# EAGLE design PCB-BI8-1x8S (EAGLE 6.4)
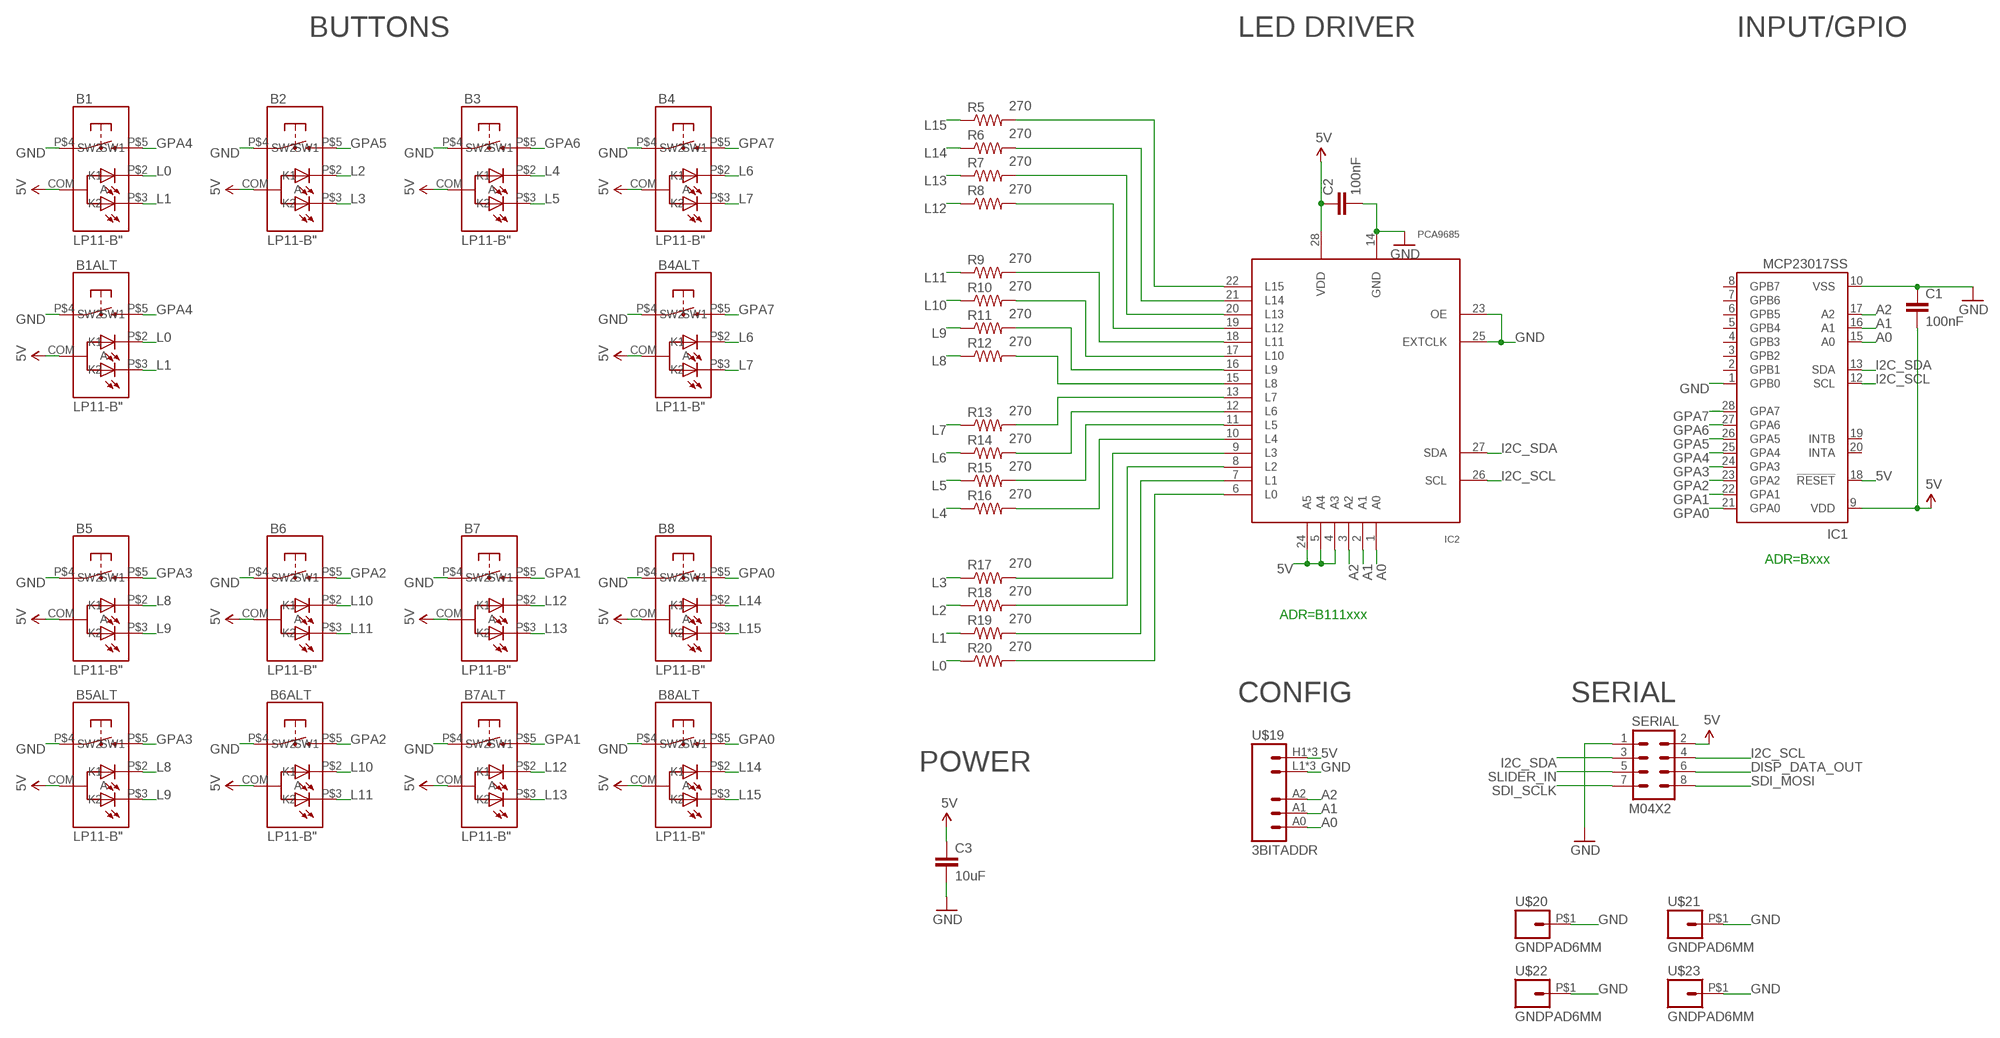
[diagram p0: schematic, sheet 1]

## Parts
B1  LP11-B"  [LP11]
B1ALT  LP11-B"  [LP11]
B2  LP11-B"  [LP11]
B3  LP11-B"  [LP11]
B4  LP11-B"  [LP11]
B4ALT  LP11-B"  [LP11]
B5  LP11-B"  [LP11]
B5ALT  LP11-B"  [LP11]
B6  LP11-B"  [LP11]
B6ALT  LP11-B"  [LP11]
B7  LP11-B"  [LP11]
B7ALT  LP11-B"  [LP11]
B8  LP11-B"  [LP11]
B8ALT  LP11-B"  [LP11]
C1  100nF  CAP0603-CAP  [0603-CAP]
C2  100nF  CAP0603-CAP  [0603-CAP]
C3  10uF  CAP0805  [0805]
IC1  MCP23017SS  [SSOP28]
IC2  PCA9685  [TSSOP28]
R5  270  RESISTOR0603-RES  [0603-RES]
R6  270  RESISTOR0603-RES  [0603-RES]
R7  270  RESISTOR0603-RES  [0603-RES]
R8  270  RESISTOR0603-RES  [0603-RES]
R9  270  RESISTOR0603-RES  [0603-RES]
R10  270  RESISTOR0603-RES  [0603-RES]
R11  270  RESISTOR0603-RES  [0603-RES]
R12  270  RESISTOR0603-RES  [0603-RES]
R13  270  RESISTOR0603-RES  [0603-RES]
R14  270  RESISTOR0603-RES  [0603-RES]
R15  270  RESISTOR0603-RES  [0603-RES]
R16  270  RESISTOR0603-RES  [0603-RES]
R17  270  RESISTOR0603-RES  [0603-RES]
R18  270  RESISTOR0603-RES  [0603-RES]
R19  270  RESISTOR0603-RES  [0603-RES]
R20  270  RESISTOR0603-RES  [0603-RES]
SERIAL  M04X2  [2X4]
U$19  3BITADDR  [3BITADDR]
U$20  GNDPAD6MM  [3.2MMPAD6MM]
U$21  GNDPAD6MM  [3.2MMPAD6MM]
U$22  GNDPAD6MM  [3.2MMPAD6MM]
U$23  GNDPAD6MM  [3.2MMPAD6MM]

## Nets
5V [Power]: B1.COM(A) B1ALT.COM(A) B2.COM(A) B3.COM(A) B4.COM(A) B4ALT.COM(A) B5.COM(A) B5ALT.COM(A) B6.COM(A) B6ALT.COM(A) B7.COM(A) B7ALT.COM(A) B8.COM(A) B8ALT.COM(A) C1.2 C2.1 C3.1 IC1.9(VDD) IC1.18(!RESET) IC2.4(A3) IC2.5(A4) IC2.24(A5) IC2.28(VDD) SERIAL.2 U$19.H1(VCC) U$19.H2(VCC) U$19.H3(VCC)
A0: IC1.15(A0) IC2.1(A0) U$19.A0
A1: IC1.16(A1) IC2.2(A1) U$19.A1
A2: IC1.17(A2) IC2.3(A2) U$19.A2
DISP_DATA_OUT: SERIAL.6
GND [Power]: B1.P$4(SW1) B1ALT.P$4(SW1) B2.P$4(SW1) B3.P$4(SW1) B4.P$4(SW1) B4ALT.P$4(SW1) B5.P$4(SW1) B5ALT.P$4(SW1) B6.P$4(SW1) B6ALT.P$4(SW1) B7.P$4(SW1) B7ALT.P$4(SW1) B8.P$4(SW1) B8ALT.P$4(SW1) C1.1 C2.2 C3.2 IC1.1(GPB0) IC1.10(VSS) IC2.14(GND) IC2.23(OE) IC2.25(EXTCLK) SERIAL.1 U$19.L1(GND) U$19.L2(GND) U$19.L3(GND) U$20.P$1 U$21.P$1 U$22.P$1 U$23.P$1
GPA0: B8.P$5(SW2) B8ALT.P$5(SW2) IC1.21(GPA0)
GPA1: B7.P$5(SW2) B7ALT.P$5(SW2) IC1.22(GPA1)
GPA2: B6.P$5(SW2) B6ALT.P$5(SW2) IC1.23(GPA2)
GPA3: B5.P$5(SW2) B5ALT.P$5(SW2) IC1.24(GPA3)
GPA4: B1.P$5(SW2) B1ALT.P$5(SW2) IC1.25(GPA4)
GPA5: B2.P$5(SW2) IC1.26(GPA5)
GPA6: B3.P$5(SW2) IC1.27(GPA6)
GPA7: B4.P$5(SW2) B4ALT.P$5(SW2) IC1.28(GPA7)
I2C_SCL: IC1.12(SCL) IC2.26(SCL) SERIAL.4
I2C_SDA: IC1.13(SDA) IC2.27(SDA) SERIAL.3
L0: B1.P$2(K1) B1ALT.P$2(K1) R20.1
L1: B1.P$3(K2) B1ALT.P$3(K2) R19.1
L2: B2.P$2(K1) R18.1
L3: B2.P$3(K2) R17.1
L4: B3.P$2(K1) R16.1
L5: B3.P$3(K2) R15.1
L6: B4.P$2(K1) B4ALT.P$2(K1) R14.1
L7: B4.P$3(K2) B4ALT.P$3(K2) R13.1
L8: B5.P$2(K1) B5ALT.P$2(K1) R12.1
L9: B5.P$3(K2) B5ALT.P$3(K2) R11.1
L10: B6.P$2(K1) B6ALT.P$2(K1) R10.1
L11: B6.P$3(K2) B6ALT.P$3(K2) R9.1
L12: B7.P$2(K1) B7ALT.P$2(K1) R8.1
L13: B7.P$3(K2) B7ALT.P$3(K2) R7.1
L14: B8.P$2(K1) B8ALT.P$2(K1) R6.1
L15: B8.P$3(K2) B8ALT.P$3(K2) R5.1
N$4: IC2.13(L7) R13.2
N$5: IC2.12(L6) R14.2
N$7: IC2.11(L5) R15.2
N$9: IC2.10(L4) R16.2
N$10: IC2.9(L3) R17.2
N$11: IC2.8(L2) R18.2
N$12: IC2.7(L1) R19.2
N$19: IC2.6(L0) R20.2
N$20: IC2.15(L8) R12.2
N$21: IC2.16(L9) R11.2
N$22: IC2.17(L10) R10.2
N$23: IC2.18(L11) R9.2
N$24: IC2.19(L12) R8.2
N$25: IC2.20(L13) R7.2
N$26: IC2.21(L14) R6.2
N$27: IC2.22(L15) R5.2
SDI_MOSI: SERIAL.8
SDI_SCLK: SERIAL.7
SLIDER_IN: SERIAL.5
Unconnected: IC1.2(GPB1) IC1.3(GPB2) IC1.4(GPB3) IC1.5(GPB4) IC1.6(GPB5) IC1.7(GPB6) IC1.8(GPB7) IC1.19(INTB) IC1.20(INTA)

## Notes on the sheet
- BUTTONS | LED DRIVER | INPUT/GPIO
- ADR=Bxxx
- ADR=B111xxx
- CONFIG | SERIAL
- POWER

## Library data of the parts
B1 B1ALT B2-B4 B4ALT B5 B5ALT B6 B6ALT B7 B7ALT B8 B8ALT = SKAARHOJ:LP11-B
C1-C3 = SparkFun:CAP: Capacitor
IC1 = microchip:MCP23017: http://ww1.microchip.com/downloads/en/DeviceDoc/21952a.pdf Source: http://ww1.microchip.com/downloads/en/DeviceDoc/21952a.pdf; MF: MICROCHIP; MPN: MCP23017-E/SS; OC_FARNELL: 1467674; OC_NEWARK: 31K2960
IC2 = wsmith:PCA9685
R5-R20 = SparkFun:RESISTOR: Resistor
SERIAL = SparkFun:M04X2
U$19 = SKAARHOJ:3BITADDR
U$20-U$23 = SKAARHOJ:GNDPAD

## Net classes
0 default: width 0.203 mm, drill 0.305 mm, clearance 0.203 mm
1 Power: width 0.305 mm, drill 0.61 mm, clearance 0.203 mm

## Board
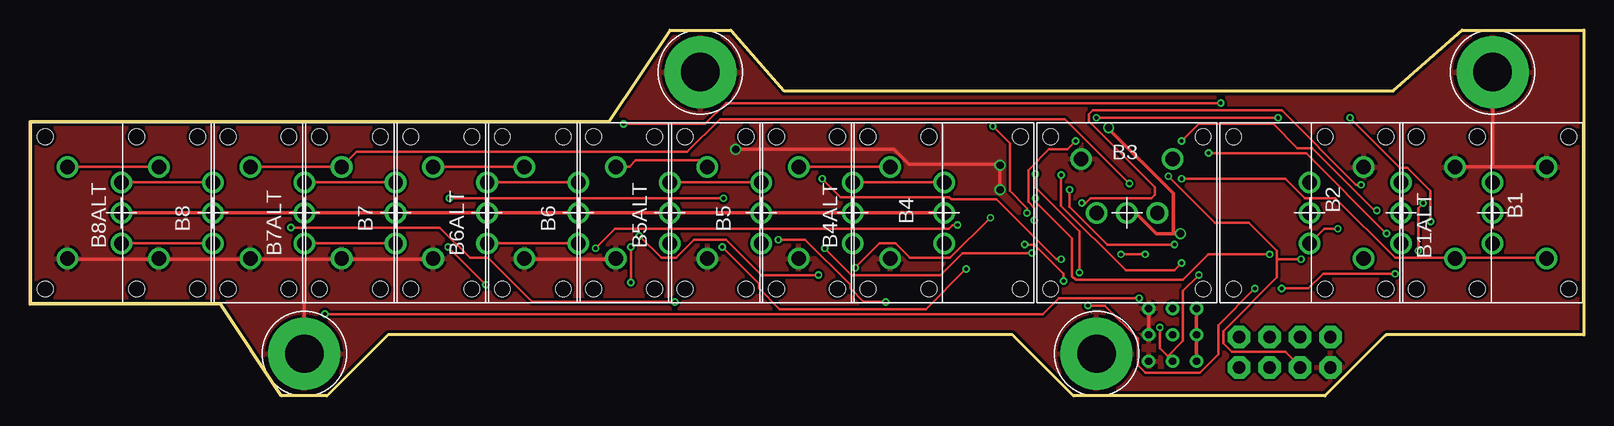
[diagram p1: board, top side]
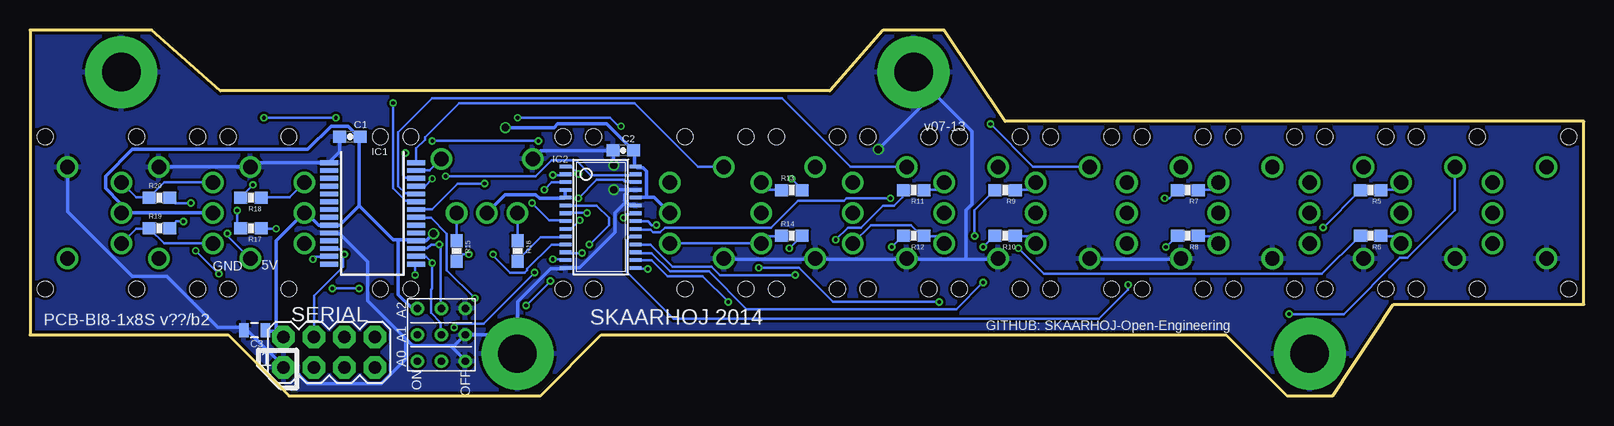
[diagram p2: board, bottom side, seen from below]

Size 129.54 x 30.48 mm. Coordinates in mm from the lower left corner, seen from the top.
Outline: 0,22.86 48.26,22.86 53.34,30.48 58.42,30.48 62.87,25.4 113.67,25.4 119.38,30.48 129.54,30.48 129.54,5.08 113.03,5.08 107.95,0 87,0 81.92,5.08 29.84,5.08 24.77,0 20.95,0 15.88,7.62 0,7.62 0,22.86
Copper layers (1*16): Top 0.035mm / dielectric 1.5mm / Bottom 0.035mm
Design rules "Fusion_eagle_rule_v1.1": minimum track width 6mil, minimum drill 12mil, track to track 6mil, track to pad 6mil, pad to pad 6mil, via to via 6mil, smd to smd 0mil, copper to edge 10mil, drill to drill 10mil, minimum pad ring 10mil, minimum via ring 6mil, stop-mask expansion 2mil, vias tented up to drill 100mil, thermal gap 10mil

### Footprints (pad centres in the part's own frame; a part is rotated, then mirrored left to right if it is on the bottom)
LP11 = drill 1.2: COM 0,0; P$2 0,2.54; P$3 0,-2.54; P$4 4.5,3.81; P$5 4.5,-3.81 | hole 1.3: -6.35,6.35; 6.35,6.35; 6.35,-6.35; -6.35,-6.35
0603-CAP = smd 1.1 x 1: 1 -0.85,0; 2 0.85,0
0805 = smd 0.8 x 1.2: 1 -0.9,0; 2 0.9,0
SSOP28 = smd 0.4 x 1.5: 1 -4.225,-3.625; 2 -3.575,-3.625; 3 -2.925,-3.625; 4 -2.275,-3.625; 5 -1.625,-3.625; 6 -0.975,-3.625; 7 -0.325,-3.625; 8 0.325,-3.625; 9 0.975,-3.625; 10 1.625,-3.625; 11 2.275,-3.625; 12 2.925,-3.625; 13 3.575,-3.625; 14 4.225,-3.625; 15 4.225,3.625; 16 3.575,3.625; 17 2.925,3.625; 18 2.275,3.625; 19 1.625,3.625; 20 0.975,3.625; 21 0.325,3.625; 22 -0.325,3.625; 23 -0.975,3.625; 24 -1.625,3.625; 25 -2.275,3.625; 26 -2.925,3.625; 27 -3.575,3.625; 28 -4.225,3.625
TSSOP28 = smd 0.305 x 0.991: 1 -4.225,-2.918; 2 -3.575,-2.918; 3 -2.925,-2.918; 4 -2.275,-2.918; 5 -1.625,-2.918; 6 -0.975,-2.918; 7 -0.325,-2.918; 8 0.325,-2.918; 9 0.975,-2.918; 10 1.625,-2.918; 11 2.275,-2.918; 12 2.925,-2.918; 13 3.575,-2.918; 14 4.225,-2.918; 15 4.225,2.918; 16 3.575,2.918; 17 2.925,2.918; 18 2.275,2.918; 19 1.625,2.918; 20 0.975,2.918; 21 0.325,2.918; 22 -0.325,2.918; 23 -0.975,2.918; 24 -1.625,2.918; 25 -2.275,2.918; 26 -2.925,2.918; 27 -3.575,2.918; 28 -4.225,2.918
0603-RES = smd 1.1 x 1: 1 -0.85,0; 2 0.85,0
2X4 = drill 1.016 pad 1.88 octagon: 1 -3.81,-1.27; 2 -3.81,1.27; 3 -1.27,-1.27; 4 -1.27,1.27; 5 1.27,-1.27; 6 1.27,1.27; 7 3.81,-1.27; 8 3.81,1.27
3BITADDR = drill 0.6: A0 -2.2,0; A1 0,0; A2 2.2,0; H1 -2.2,2; H2 0,2; H3 2.2,2; L1 -2.2,-2; L2 0,-2; L3 2.2,-2
3.2MMPAD6MM = drill 3.2 pad 6: P$1 0,0

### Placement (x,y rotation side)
B1  121.92,15.24 0 top
B1ALT  114.3,15.24 0 top
B2  106.68,15.24 0 top
B3  91.44,15.24 90 top
B4  76.2,15.24 180 top
B4ALT  68.58,15.24 180 top
B5  60.96,15.24 180 top
B5ALT  53.34,15.24 180 top
B6  45.72,15.24 180 top
B6ALT  38.1,15.24 180 top
B7  30.48,15.24 180 top
B7ALT  22.86,15.24 180 top
B8  15.24,15.24 180 top
B8ALT  7.62,15.24 180 top
C1  102.87,21.59 0 bottom
C2  80.09,20.45 180 bottom
C3  110.82,5.46 180 bottom
IC1  100.99,15.19 270 bottom
IC2  81.97,14.88 270 bottom
R5  17.78,17.14 180 bottom
R6  17.78,13.34 180 bottom
R7  33.02,17.14 180 bottom
R8  33.02,13.34 180 bottom
R9  48.26,17.14 180 bottom
R10  48.26,13.34 180 bottom
R11  55.88,17.14 180 bottom
R12  55.88,13.34 180 bottom
R13  66.04,17.14 0 bottom
R14  66.04,13.34 0 bottom
R15  93.98,12.06 270 bottom
R16  88.9,12.06 270 bottom
R17  111.12,13.97 180 bottom
R18  111.12,16.51 180 bottom
R19  118.75,13.97 0 bottom
R20  118.75,16.51 0 bottom
SERIAL  104.6,3.63 0 bottom
U$19  95.25,5.08 90 bottom
U$20  22.86,3.5 0 top
U$21  55.88,26.98 0 top
U$22  121.92,26.98 0 top
U$23  88.9,3.5 0 top

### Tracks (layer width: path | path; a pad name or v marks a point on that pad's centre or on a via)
5V  (via drill 0.61)
  Top 0.305: U$19.H1 97.23,2.95 97.23,5.08 U$19.H2 97.23,5.18 97.23,7.21 U$19.H3 | B3.COM 92.15,15.24 93.88,13.51 95.3,13.51 | v95.91,13.51 95.3,13.51 | B8ALT.COM B8.COM B7ALT.COM B7.COM B6ALT.COM B6.COM B5ALT.COM B5.COM B4ALT.COM B4.COM | 95.3,13.51 95.3,16.87 89.92,22.25 v89.92,22.35
  Bottom 0.305: B1ALT.COM B1.COM 122.02,15.34 122.02,16.05 123.24,17.27 123.24,18.29 121.01,20.52 106.38,20.52 104.44,22.45 103.02,22.45 102.21,21.64 C1.2 102.11,21.54 102.11,15.85 | IC2.4 84.94,17.07 84.94,16.56 IC2.5 85.04,16.46 87.07,16.46 87.38,16.76 89.92,16.76 B3.COM | C3.1 109.83,5.38 108.81,5.38 108.41,4.98 SERIAL.2 109.02,5.49 109.02,12.9 B2.COM 106.48,15.24 105.46,14.22 104.75,14.22 IC1.9 104.55,14.22 103.73,14.22 102.11,15.85 | 98.86,13.01 99.26,13.01 102.11,15.85 | 98.86,13.01 97.43,13.01 IC1.18 97.23,12.9 96.52,12.9 v95.91,13.51 | 98.86,13.01 98.86,8.43 97.74,7.32 97.33,7.32 U$19.H3 | 78.13,16.56 77.52,16.56 B4.COM | 78.13,16.56 79.05,16.56 IC2.24 | 78.13,16.56 78.13,18.69 78.44,19 78.94,19 IC2.28 79.15,19.2 79.15,20.42 C2.1 79.35,20.52 81.48,22.66 85.55,22.66 85.85,22.35 v89.92,22.35
A0  (via drill 0.3)
  Top 0.203: v83.82,18.49 83.82,17.37 87.48,13.72 v87.48,10.26 | v94.18,5.69 94.18,3.96 94.84,3.3 | 94.84,3.3 95.2,2.95 U$19.A0 | v97.43,10.06 96.11,8.74 96.11,4.57 94.84,3.3
  Bottom 0.203: v83.82,18.49 84.43,19.1 84.84,19.1 IC2.1 | v87.48,10.26 91.75,5.99 93.88,5.99 v94.18,5.69 | v97.43,10.06 97.43,10.87 IC1.15
A1  (via drill 0.3)
  Top 0.203: v85.95,18.39 85.95,15.85 91.34,10.46 95.4,10.46 v96.01,11.07
  Bottom 0.203: v85.95,18.39 84.94,18.39 IC2.2 | IC1.16 97.33,11.58 96.52,11.58 v96.01,11.07 96.01,8.94 96.11,8.84 96.11,6.91 95.3,6.1 95.3,5.08 U$19.A1
A2  (via drill 0.3)
  Top 0.203: v86.67,17.17 86.67,15.75 89.81,12.6 v95.4,12.6
  Bottom 0.203: v86.67,17.17 86.06,17.78 84.94,17.78 IC2.3 | IC1.17 97.33,12.29 96.42,12.29 96.11,12.6 v95.4,12.6 95.3,12.5 95.3,7.32 U$19.A2
GND  (via drill 0.61)
  Top 0.305: 121.92,19.1 126.39,19.1 B1.P$4 | 121.92,19.1 118.87,19.1 B1ALT.P$4 | U$22.P$1 121.92,19.1 | U$19.L3 93.27,7.21 93.27,5.08 U$19.L2 | v80.87,17.17 v80.87,19.2 80.77,19.3 73.25,19.3 72.03,20.52 v58.83,20.52 | B6.P$4 41.25,11.38 48.77,11.38 B5ALT.P$4 | B8ALT.P$4 3.15,11.38 10.67,11.38 B8.P$4 10.87,11.38 18.29,11.38 B7ALT.P$4 18.49,11.38 22.86,11.38 | 22.86,11.38 25.91,11.38 B7.P$4 26.11,11.38 33.53,11.38 B6ALT.P$4 | 22.86,11.38 U$20.P$1
  Bottom 0.305: C1.1 103.73,21.54 103.73,20.32 104.55,19.51 IC1.1 104.75,19.41 110.85,19.41 111.15,19.1 B2.P$4 111.25,19.1 118.77,19.1 B1ALT.P$4 | 98.15,4.67 97.64,4.17 94.39,4.17 | 98.15,4.67 101.4,7.92 101.4,11.18 103.73,13.51 104.55,13.51 IC1.10 | 94.39,4.17 94.18,4.17 93.27,5.08 U$19.L2 89,5.08 U$23.P$1 88.9,7.82 86.16,10.57 84.94,10.57 IC2.14 84.73,10.67 83.72,10.67 80.77,13.61 80.77,15.24 79.86,16.15 | U$19.L1 93.27,2.95 94.39,4.06 94.39,4.17 | 98.15,4.67 98.25,4.57 98.25,3.05 100.28,1.02 106.38,1.02 107.7,2.34 108.31,2.34 SERIAL.1 108.41,2.44 111.35,5.38 111.66,5.38 C3.2 111.86,5.49 112.06,5.69 113.89,5.69 118.16,9.96 121.01,9.96 126.39,15.34 126.39,19 B1.P$4 | B3.P$4 87.58,19.81 86.97,20.42 80.97,20.42 C2.2 80.87,20.32 v80.87,19.2 | 79.86,16.15 79.96,16.26 79.96,16.76 79.65,17.07 | 79.86,16.15 79.65,15.95 79.15,15.95 IC2.23 | 79.65,17.07 79.55,17.17 79.15,17.17 IC2.25 | v80.87,17.17 79.76,17.17 79.65,17.07 | B4.P$4 71.63,11.38 64.21,11.38 B4ALT.P$4 64.01,11.38 56.49,11.38 B5.P$4 56.39,11.38 51.51,11.38 | B6.P$4 41.15,11.38 33.63,11.38 B6ALT.P$4 | 51.51,11.38 48.87,11.38 B5ALT.P$4 | 51.51,11.38 51.51,15.44 51,15.95 51,22.05 55.88,26.92 U$21.P$1 54.25,25.09 v58.83,20.52
  pour Top: 0,0 129.54,0 129.54,30.48 0,30.48
  pour Bottom: 0,0 129.54,0 129.54,30.48 0,30.48
GPA0  (via drill 0.3)
  Top 0.203: v92.46,8.13 85.75,8.13 84.43,6.81 v24.59,6.81 | B8ALT.P$5 3.15,19.1 10.67,19.1 B8.P$5
  Bottom 0.203: v92.46,8.13 94.79,10.46 94.79,13.51 96.11,14.83 97.33,14.83 IC1.21 | v24.59,6.81 20.02,6.81 15.34,11.48 14.73,11.48 10.77,15.44 10.77,19 B8.P$5
GPA1  (via drill 0.3)
  Top 0.203: v91.64,17.68 86.26,23.06 57.51,23.06 54.76,20.32 27.23,20.32 26.01,19.1 B7.P$5 25.91,19.1 18.39,19.1 B7ALT.P$5
  Bottom 0.203: v91.64,17.68 93.88,17.68 96.01,15.54 97.33,15.54 IC1.22
GPA2  (via drill 0.3)
  Top 0.203: v99.26,24.38 58.01,24.38 56.29,22.66 v49.48,22.66 | B6ALT.P$5 33.63,19.1 41.15,19.1 B6.P$5
  Bottom 0.203: v99.26,24.38 99.26,17.27 98.25,16.26 97.43,16.26 IC1.23 | v49.48,22.66 45.92,19.1 41.25,19.1 B6.P$5
GPA3
  Top 0.203: B5ALT.P$5 48.87,19.1 49.99,19.1 50.49,19.61 55.88,19.61 56.39,19.1 B5.P$5
  Bottom 0.203: IC1.24 97.43,16.87 98.25,16.87 98.86,17.48 98.86,21.95 96.01,24.79 66.85,24.79 61.16,19.1 56.49,19.1 B5.P$5
GPA4  (via drill 0.3)
  Top 0.203: v96.01,18.09 104.65,18.09 106.27,16.46 108.81,16.46 113.79,11.48 118.77,11.48 B1ALT.P$5 118.87,11.48 126.39,11.48 B1.P$5
  Bottom 0.203: v96.01,18.09 96.62,17.48 97.33,17.48 IC1.25
GPA5  (via drill 0.3)
  Top 0.203: v98.25,20.22 106.38,20.22 v113.08,13.51
  Bottom 0.203: v98.25,20.22 98.45,20.02 98.45,18.39 98.25,18.19 97.43,18.19 IC1.26 | v113.08,13.51 113.08,13.31 111.25,11.48 B2.P$5
GPA6
  Bottom 0.203: IC1.27 97.33,18.8 96.22,18.8 95.3,19.71 B3.P$5
GPA7
  Top 0.203: B4ALT.P$5 64.11,19.1 71.63,19.1 B4.P$5
  Bottom 0.203: IC1.28 97.33,19.51 97.33,20.62 96.62,21.34 96.62,21.54 93.78,24.38 79.15,24.38 73.86,19.1 71.73,19.1 B4.P$5
I2C_SCL  (via drill 0.3)
  Top 0.203: v83.82,16.46 83.82,16.15 86.87,13.11 86.87,9.96 87.17,9.65 96.11,9.65 98.25,11.79 v103.33,11.79
  Bottom 0.203: v83.82,16.46 82.3,17.98 80.06,17.98 79.96,17.88 79.15,17.88 IC2.26 | IC1.12 104.55,12.19 103.73,12.19 v103.33,11.79 103.43,11.79 103.43,10.77 105.87,8.33 SERIAL.4
I2C_SDA  (via drill 0.3)
  Top 0.203: v94.89,18.29 98.75,14.43 101.6,14.43 103.94,12.09 103.94,11.38 | 103.94,11.38 103.94,9.86 99.47,5.38 99.47,4.37 100.18,3.66 104.65,3.66 105.87,2.44 SERIAL.3 | 103.94,11.38 v105.97,11.38
  Bottom 0.203: v94.89,18.29 87.38,18.29 86.06,19.61 84.02,19.61 82.8,18.39 79.15,18.39 IC2.27 | v105.97,11.38 105.77,11.58 104.65,11.58 IC1.13
L0
  Bottom 0.203: B1.P$2 120.7,16.56 119.69,16.56 R20.1 119.58,16.56 118.36,17.78 B1ALT.P$2
L1
  Bottom 0.203: B1.P$3 120.7,13.92 119.69,13.92 R19.1 119.58,13.92 118.36,12.7 B1ALT.P$3
L2
  Bottom 0.203: B2.P$2 107.9,16.56 110.24,16.56 R18.1
L3  (via drill 0.3)
  Top 0.203: v109.02,13.92 107.9,13.92 B2.P$3
  Bottom 0.203: v109.02,13.92 110.24,13.92 R17.1
L4
  Bottom 0.203: B3.P$2 R16.1
L5
  Bottom 0.203: B3.P$3 R15.1
L6
  Bottom 0.203: R14.1 66.95,13.31 67.97,13.31 B4ALT.P$2 B4.P$2
L7
  Top 0.203: B4.P$3 B4ALT.P$3
  Bottom 0.203: B4ALT.P$3 67.97,17.17 66.95,17.17 R13.1
L8
  Bottom 0.203: B5ALT.P$2 53.95,13.31 54.97,13.31 R12.1 55.07,13.41 55.27,13.41 56.08,14.22 59.44,14.22 B5.P$2
L9
  Top 0.203: B5.P$3 B5ALT.P$3
  Bottom 0.203: B5ALT.P$3 53.95,17.17 54.97,17.17 R11.1
L10
  Top 0.203: B6.P$2 B6ALT.P$2
  Bottom 0.203: B6.P$2 46.33,13.31 47.35,13.31 R10.1
L11
  Top 0.203: B6.P$3 B6ALT.P$3
  Bottom 0.203: B6.P$3 46.33,17.17 47.35,17.17 R9.1
L12
  Top 0.203: B7.P$2 B7ALT.P$2
  Bottom 0.203: B7.P$2 31.09,13.31 32.11,13.31 R8.1
L13
  Top 0.203: B7.P$3 B7ALT.P$3
  Bottom 0.203: B7.P$3 31.09,17.17 32.11,17.17 R7.1
L14
  Top 0.203: B8.P$2 B8ALT.P$2
  Bottom 0.203: B8.P$2 15.85,13.31 16.87,13.31 R6.1
L15
  Top 0.203: B8.P$3 B8ALT.P$3
  Bottom 0.203: B8.P$3 15.85,17.17 16.87,17.17 R5.1
N$4  (via drill 0.3)
  Top 0.203: v85.95,11.38 85.55,11.38 80.57,16.36 76.81,16.36 76.61,16.56 67.56,16.56 v66.04,18.09
  Bottom 0.203: v85.95,11.38 84.94,11.38 IC2.13 | v66.04,18.09 65.13,17.17 R13.2
N$5  (via drill 0.3)
  Top 0.203: v83.52,11.89 77.72,11.89 75.89,10.06 68.48,10.06 v66.24,12.29
  Bottom 0.203: v83.52,11.89 84.84,11.89 IC2.12 | v66.24,12.29 65.23,13.31 R14.2
N$7  (via drill 0.3)
  Top 0.203: v92.96,11.79 v90.93,11.79
  Bottom 0.203: v90.93,11.79 90.93,11.68 89.51,10.26 88.29,10.26 88.09,10.46 88.09,10.57 86.06,12.6 84.94,12.6 IC2.11 | v92.96,11.79 93.47,11.79 93.98,11.28 R15.2
N$9
  Bottom 0.203: IC2.10 84.94,13.21 86.97,13.21 88.9,11.28 R16.2
N$10  (via drill 0.3)
  Top 0.203: v83.72,14.63 83.72,15.65 83.21,16.15 83.21,18.8 84.94,20.52 86.46,20.52 v87.17,21.23 | v96.01,21.23 97.43,22.66 103.63,22.66 105.66,20.62 106.88,20.62 112.06,15.44 v112.27,15.44
  Bottom 0.203: v83.72,14.63 84.43,13.92 84.84,13.92 IC2.9 | v96.01,21.23 v87.17,21.23 | v112.27,15.44 112.27,14.22 112.06,14.02 R17.2
N$11  (via drill 0.3)
  Top 0.203: v87.68,16.05 87.99,16.05 88.39,16.46 93.47,16.46 93.78,16.76 93.78,17.37 88.29,22.86 88.29,23.47 88.59,23.77 104.34,23.77 110.54,17.58 v110.95,17.58
  Bottom 0.203: v87.68,16.05 86.26,14.63 84.94,14.63 IC2.8 | v110.95,17.58 111.96,16.56 R18.2
N$12  (via drill 0.3)
  Top 0.203: v83.11,15.24 83.11,15.65 81.69,17.07 81.69,21.03 v80.26,22.45 | v104.04,23.16 v88.9,23.16 | v110.03,23.16 114.2,19 114.81,19 116.74,17.07 v116.74,14.53
  Bottom 0.203: v83.11,15.24 84.84,15.24 IC2.7 | v80.26,22.45 80.47,22.45 81.18,23.16 v88.9,23.16 | v110.03,23.16 v104.04,23.16 | v116.74,14.53 117.35,14.53 117.86,14.02 R19.2
N$19  (via drill 0.3)
  Top 0.203: v82.91,12.6 83.72,12.6 86.16,10.16 v86.16,9.55 | v88.19,7.52 89.61,7.52 92.35,4.78 92.35,2.54 92.96,1.93 97.54,1.93 99.06,3.45 99.06,5.89 v102.11,8.94 | v104.34,8.94 106.58,8.94 107.8,10.16 v113.79,10.16 | v115.72,12.09 115.72,15.65 v116.13,16.05
  Bottom 0.203: v82.91,12.6 81.28,14.22 81.28,14.83 82.3,15.85 84.84,15.85 IC2.6 | v88.19,7.52 v86.16,9.55 | v104.34,8.94 v102.11,8.94 | v115.72,12.09 v113.79,10.16 | v116.13,16.05 117.45,16.05 117.86,16.46 R20.2
N$20  (via drill 0.3)
  Top 0.203: v78.03,10.57 74.68,7.21 62.48,7.21 60.76,8.94 60.76,9.35 v57.71,12.39
  Bottom 0.203: v78.03,10.57 79.05,10.57 IC2.15 | v57.71,12.39 56.79,13.31 R12.2
N$21  (via drill 0.3)
  Top 0.203: v71.32,7.82 69.49,7.82 68.38,8.94 68.38,9.25 64.62,13.01 v62.38,13.01
  Bottom 0.203: v71.32,7.82 73.46,9.96 76.4,9.96 77.72,11.28 79.05,11.28 IC2.16 | v62.38,13.01 61.37,14.02 60.25,14.02 58.42,15.85 57.51,15.85 56.79,16.56 56.79,17.07 R11.2
N$22  (via drill 0.3)
  Top 0.203: v50.09,12.39 v50.09,9.45
  Bottom 0.203: v50.09,9.45 52.32,7.21 69.8,7.21 72.95,10.36 76.2,10.36 77.72,11.89 79.05,11.89 IC2.17 | v50.09,12.39 49.17,13.31 R10.2
N$23  (via drill 0.3)
  Top 0.203: v65.73,10.06 60.96,10.06 58.01,13.01 55.37,13.01 53.85,11.48 52.63,11.48 v50.8,13.31
  Bottom 0.203: v65.73,10.06 72.03,10.06 72.75,10.77 76,10.77 77.83,12.6 79.05,12.6 IC2.18 | v50.8,13.31 50.8,15.44 49.17,17.07 R9.2
N$24  (via drill 0.3)
  Top 0.203: v34.85,12.39 v38,9.25
  Bottom 0.203: v38,9.25 38,8.84 40.44,6.4 75.89,6.4 79.86,10.36 79.86,12.9 79.55,13.21 79.15,13.21 IC2.19 | v34.85,12.39 33.93,13.31 R8.2
N$25  (via drill 0.3)
  Top 0.203: v34.95,16.46 v57.81,16.46
  Bottom 0.203: v57.81,16.46 61.47,16.46 61.67,16.26 65.53,16.26 67.77,14.02 76.61,14.02 77.01,13.61 77.62,13.61 77.83,13.82 79.05,13.82 IC2.20 | v34.95,16.46 34.54,16.46 33.93,17.07 R7.2
N$26  (via drill 0.3)
  Top 0.203: v77.32,14.22 76.91,14.22 76.61,13.92 48.77,13.92 v47.14,12.29
  Bottom 0.203: v77.32,14.22 77.72,14.22 78.03,14.53 79.05,14.53 IC2.21 | v47.14,12.29 45.01,10.16 21.84,10.16 18.69,13.31 R6.2
N$27  (via drill 0.3)
  Top 0.203: v80.06,14.83 76.71,11.48 73.36,11.48 72.14,12.7 70.81,12.7 v68.78,10.67 | v53.75,7.82 41.86,7.82 38.2,11.48 36.68,11.48 34.14,14.02 v21.74,14.02
  Bottom 0.203: v80.06,14.83 79.76,15.14 79.15,15.14 IC2.22 | v68.78,10.67 65.43,10.67 62.59,7.82 v53.75,7.82 | v21.74,14.02 18.69,17.07 R5.2

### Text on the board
_bsilk: v07-13 | GND | 5V | SKAARHOJ 2014 | PCB-BI8-1x8S v??/b2 | GITHUB: SKAARHOJ-Open-Engineering | 1

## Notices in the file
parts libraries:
SparkFun: Licensing: CC v3.0 Share-Alike You are welcome to use this library for commercial purposes.
